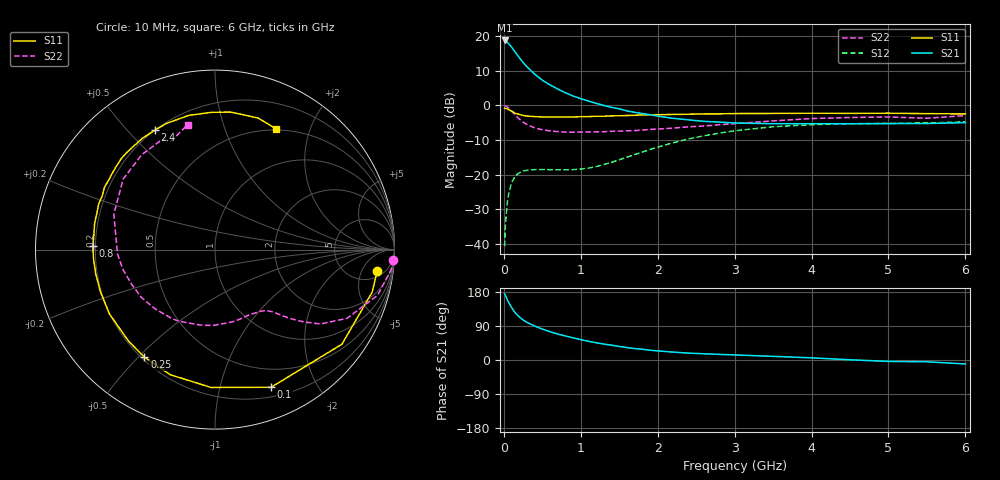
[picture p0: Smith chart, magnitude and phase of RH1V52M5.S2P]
! SIEMENS Small Signal Semiconductors
! BFR106
! Si NPN RF Bipolar Junction Transistor in SOT23
! VCE = 1.5 V  IC = 2.5 mA
! Common Emitter S-Parameters:  August  1996
# GHz  S  MA  R  50
!  f  S11  S21  S12  S22
! GHz  MAG  ANG  MAG  ANG  MAG  ANG  MAG  ANG
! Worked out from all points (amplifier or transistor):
!   36 points, 10 MHz to 6 GHz, reference 50 ohm
!   highest |S21| = 18.8 dB at 10 MHz (marker M1)
!   |S21| within 3 dB of that: start of sweep to 135.1 MHz
!   unconditionally stable (mu >= 1): 733 MHz to 2.522 GHz; 2.776 GHz to end of sweep
!   at 250 MHz: K = 0.36, MSG = 15.7 dB, |S12| = -19.0 dB
!   at 1.4 GHz: K = 1.27, MAG = 4.8 dB, |S12| = -16.5 dB
!   at 6 GHz: K = 1.03, MAG = -1.1 dB, |S12| = -4.8 dB
!   S11 on the Smith chart (normalised r, x): 10 MHz: 7, -10; 100 MHz: 0.30, -1.45; 250 MHz: 0.21, -0.52; 800 MHz: 0.19, +0.01; 2.4 GHz: 0.20, +0.60; 6 GHz: 0.48, +1.51
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0.01  0.9113 -7.6  8.697 174.6  0.0092 87.1  0.9955 -3.3
0.02  0.9074 -15.1  8.681 170.6  0.0185 83.2  0.9875 -6.6
0.05  0.882 -36.7  8.104 156.6  0.0446 70.0  0.9407 -15.7
0.1  0.8283 -67.8  6.994 138.7  0.0771 54.8  0.8294 -27.5
0.15  0.7684 -91.6  5.832 123.8  0.0954 43.5  0.7188 -35.2
0.2  0.7404 -109.6  4.918 113.9  0.106 36.5  0.6374 -39.2
0.25  0.7168 -123.3  4.179 105.5  0.1123 31.6  0.5725 -42.3
0.3  0.7011 -133.5  3.615 99.4  0.1153 28.7  0.5298 -44.3
0.4  0.6888 -148.7  2.836 89.7  0.1179 25.1  0.4735 -47.1
0.5  0.6803 -159.8  2.314 81.5  0.1181 23.8  0.444 -49.9
0.6  0.678 -168.6  1.979 74.6  0.1176 24.5  0.4277 -53.4
0.8  0.6806 178.4  1.524 63.4  0.1169 28.9  0.4112 -61.6
1.1  0.689 162.7  1.154 49.3  0.1239 40.5  0.4134 -75.7
1.6  0.7138 143.0  0.832 32.7  0.1785 55.7  0.429 -102.1
2.2  0.7405 123.1  0.65 20.8  0.288 54.9  0.4696 -135.4
2.4  0.7448 116.8  0.618 18.2  0.3271 51.8  0.4895 -147.1
3  0.7619 101.1  0.557 13.4  0.4295 39.7  0.5438 -177.5
3.5  0.7652 91.3  0.543 9.6  0.4909 29.0  0.5972 160.7
4.5  0.7676 77.6  0.543 0.6  0.5419 10.2  0.6679 127.7
5  0.7713 71.9  0.545 -3.8  0.5501 3.1  0.6802 115.8
5.5  0.7596 67.0  0.547 -4.7  0.5569 -0.1  0.6519 111.9
6  0.7538 63.3  0.563 -10.5  0.5782 -7.4  0.7121 102.4
